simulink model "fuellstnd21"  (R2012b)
settings: Solver=ode45  StartTime=0.0  StopTime=10.0  RelTol=1e-3
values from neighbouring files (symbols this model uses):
  A1 = 0.02    [fuellstnd_1.m]    (also in fuellstnd_2.m; fuellstnd_21.m; fuellstnd_3.m; fuellstnd_31.m)
  A12 = 0.005    [fuellstnd_1.m]    (also in fuellstnd_2.m; fuellstnd_21.m; fuellstnd_3.m; fuellstnd_31.m)
  A2 = A1    (= 0.02)    [fuellstnd_1.m]    (also in fuellstnd_2.m; fuellstnd_21.m; fuellstnd_3.m; fuellstnd_31.m)
  A23 = A12    (= 0.005)    [fuellstnd_1.m]    (also in fuellstnd_2.m; fuellstnd_21.m; fuellstnd_3.m; fuellstnd_31.m)
  A3 = A1    (= 0.02)    [fuellstnd_1.m]    (also in fuellstnd_2.m; fuellstnd_21.m; fuellstnd_3.m; fuellstnd_31.m)
  A30 = A12    (= 0.005)    [fuellstnd_1.m]    (also in fuellstnd_2.m; fuellstnd_21.m; fuellstnd_3.m; fuellstnd_31.m)
  g = 9.89    [fuellstnd_1.m]    (also in fuellstnd_2.m; fuellstnd_21.m; fuellstnd_3.m; fuellstnd_31.m)
  h10 = 0.0    (= 0)    [fuellstnd_1.m]    (also in fuellstnd_2.m; fuellstnd_21.m; fuellstnd_3.m; fuellstnd_31.m)
  h20 = h10    (= 0)    [fuellstnd_1.m]    (also in fuellstnd_2.m; fuellstnd_21.m; fuellstnd_3.m; fuellstnd_31.m)
  h30 = h10    (= 0)    [fuellstnd_1.m]    (also in fuellstnd_2.m; fuellstnd_21.m; fuellstnd_3.m; fuellstnd_31.m)
  Tp = 1    [fuellstnd_2.m]    (also in fuellstnd_21.m = 0.1; fuellstnd_3.m = 0.1; fuellstnd_31.m = 0.01; regulator_1.m = 5)
  Usoll = 0.4,    [fuellstnd_2.m]    (also in fuellstnd_21.m = 0.2,; fuellstnd_3.m = 0.2,; fuellstnd_31.m = 0.2,)
undefined symbols (not defined in the file or in its folder): sgn

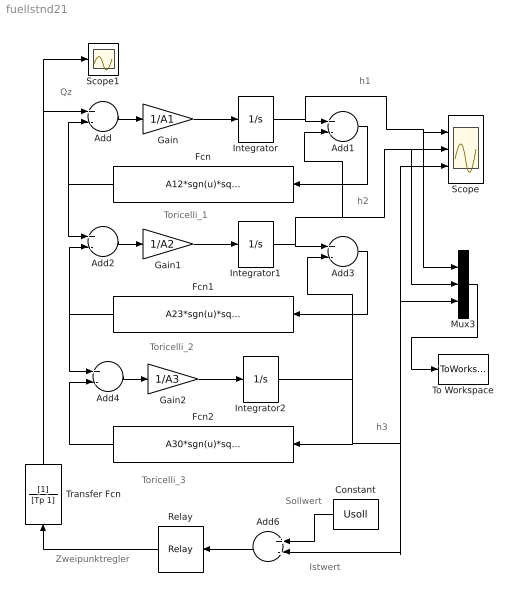
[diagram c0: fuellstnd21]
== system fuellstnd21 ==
  note: Zweipunktregler
  note: Toricelli_3
  note: Istwert
  note: Sollwert
  note: h3
  note: h2
  note: h1
  note: Toricelli_2
  note: Toricelli_1
  note: Qz
  Add{,1..4,6} (6 alike) : Sum  Inputs=+-
  Constant : Constant  Value=Usoll
  Fcn : Fcn  Expr=A12*sgn(u)*sqrt(2*g*abs(u))
  Fcn1 : Fcn  Expr=A23*sgn(u)*sqrt(2*g*abs(u))
  Fcn2 : Fcn  Expr=A30*sgn(u)*sqrt(2*g*abs(u))
  Gain : Gain  Gain=1/A1
  Gain1 : Gain  Gain=1/A2
  Gain2 : Gain  Gain=1/A3
  Integrator : Integrator  InitialCondition=h10
  Integrator1 : Integrator  InitialCondition=h20
  Integrator2 : Integrator  InitialCondition=h30
  Mux3 : Mux  Inputs=3
  Relay : Relay  OnOutputValue=Qp
  Scope : Scope  NumInputPorts=3
  Scope1 : Scope
  To Workspace : ToWorkspace  VariableName=y  SampleTime=-1  SaveFormat=Structure With Time
  Transfer Fcn : TransferFcn  Denominator=[Tp 1]
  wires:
  Add/1 -> Gain/1
  Gain/1 -> Integrator/1
  Add1/1 -> Fcn/1
  Fcn/1 -> Add/2, Add2/1
  Add2/1 -> Gain1/1
  Gain1/1 -> Integrator1/1
  Fcn1/1 -> Add4/1, Add2/2
  Add4/1 -> Gain2/1
  Gain2/1 -> Integrator2/1
  Fcn2/1 -> Add4/2
  Integrator2/1 -> Fcn2/1, Mux3/3, Scope/3, Add6/2, Add3/2
  Mux3/1 -> To Workspace/1
  Relay/1 -> Transfer Fcn/1
  Integrator1/1 -> Mux3/2, Scope/2, Add1/2, Add3/1
  Integrator/1 -> Mux3/1, Scope/1, Add1/1
  Add6/1 -> Relay/1
  Constant/1 -> Add6/1
  Add3/1 -> Fcn1/1
  Transfer Fcn/1 -> Scope1/1, Add/1
